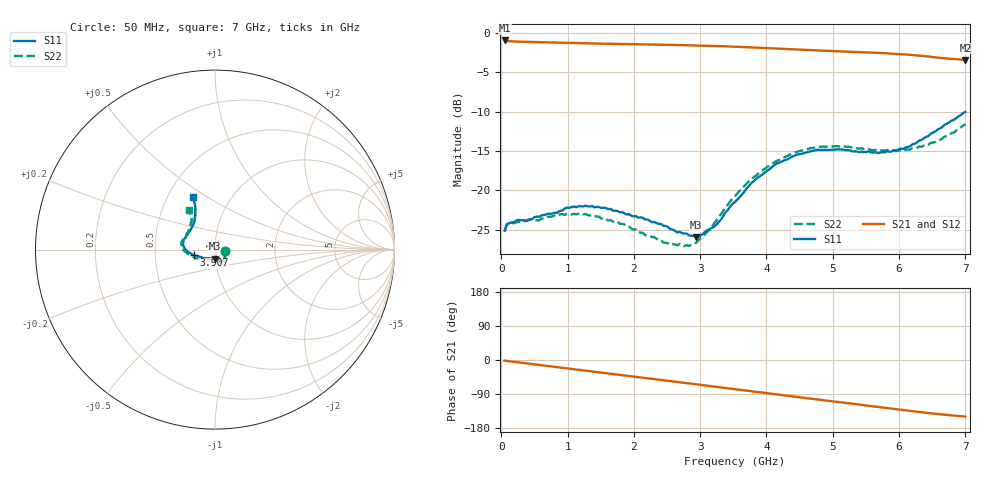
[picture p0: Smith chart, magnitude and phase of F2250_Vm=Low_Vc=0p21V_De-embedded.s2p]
! Integrated Device Technology
! Corporate Headquarters
! 6024 Silver Creek Valley Road
! San Jose, CA 95138  USA
! Phone:  1-408-284-8200
! Toll Free:  1-800-223-1366
! Webpage:  http://www.idt.com/
! Timing and RF Division
! 515 Groton Road, Suite 102
! Westford, MA 01886-6024
! Device:  F2250
! Description: Voltage Variable RF Attenuator
! Frequency:  50.0 -  6000.00 MHz
! Package:  3x3 mm Thin QFN Plastic Package: 16 pin
! Ports:  2 RF, 3 DC
!  Pin  1  = GND
!  Pin  2  = NC
!  Pin  3  = RF1  = Port 1
!  Pin  4  = NC
!  Pin  5  = GND
!  Pin  6  = GND
!  Pin  7  = GND
!  Pin  8  = GND
!  Pin  9  = NC
!  Pin 10  = RF2  = Port 2
!  Pin 11  = NC
!  Pin 12  = GND
!  Pin 13  = GND
!  Pin 14  = VCNTRL
!  Pin 15  = VDD
!  Pin 16  = VMODE
! Vcntrl:  0.210 Volts
! Vmode:  +0.000 Volts
! Vdd:  +3.30  Volts
! Current:  1.105 mA
! Data:  The device was measured on a the F2250 evaluation board which has
!  individual transmission lines to the RF pins.  Data was collected
!  using a calibrated network analyzer.  The evaluation board was
!  de-embedded using a TRL calibration technique.
!  The reference plane is the edge of the package pin.
! Misc:  SN 10
!  Action Tracker AT0258
! Date Measured:  2014-11-26
! Date:  2015-10-15  MJV
! Note:
!  Integrated Device Technology supplies this data as a sample of measured
!  data at the package pin for this product.  Your particular data for this
!  product may vary.
!  Data was taken at 25 degrees C.
!  Integrated Device Technology reserves the right to change this data at anytime.
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# GHz S dB R 50
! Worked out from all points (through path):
!   201 points, 50 MHz to 7 GHz, reference 50 ohm
!   highest |S21| = -0.93 dB at 50 MHz (marker M1); lowest = -3.4 dB at 7 GHz (marker M2)
!   group delay of S21, straight-line fit = 60 ps
!   lowest |S11| = -26.0 dB at 2.934 GHz (marker M3), VSWR 1.11, Z = 49.5 - j4.99 ohm
!   |S11| at or under -10 dB: start of sweep to end of sweep
!   |S22| runs from -27.1 to -11.6 dB; largest |S21 - S12| = 0.00027
!   S11 on the Smith chart (normalised r, x): 50 MHz: 1.12, -0.02; 3.907 GHz: 0.79, -0.05; 7 GHz: 0.67, +0.43
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0.05  -25.11 -9.7  -0.93 -1.8  -0.93 -1.8  -25.23 -10.1
0.08475  -24.29 -9.6  -1.00 -2.5  -0.99 -2.5  -24.34 -9.4
0.15425  -24.07 -11.9  -1.04 -4.0  -1.04 -4.0  -24.11 -11.0
0.57125  -23.35 -30.0  -1.14 -13.1  -1.14 -13.1  -23.82 -30.4
0.884  -22.62 -45.9  -1.21 -19.9  -1.20 -19.9  -23.05 -46.9
1.2315  -22.06 -56.1  -1.28 -27.4  -1.28 -27.4  -23.05 -59.7
1.75275  -22.62 -62.8  -1.37 -38.4  -1.37 -38.4  -23.95 -66.7
2.37825  -24.26 -63.6  -1.46 -51.8  -1.46 -51.8  -26.30 -67.8
2.552  -24.95 -67.8  -1.49 -55.6  -1.49 -55.6  -26.96 -73.3
2.83  -25.72 -83.3  -1.54 -61.7  -1.54 -61.7  -27.08 -92.7
2.93425  -25.97 -92.5  -1.56 -64.0  -1.56 -64.0  -26.70 -101.5
3.21225  -24.62 -122.1  -1.63 -70.1  -1.63 -70.1  -24.17 -127.6
3.525  -21.47 -148.4  -1.72 -77.1  -1.72 -77.1  -20.72 -146.4
3.76825  -19.10 -161.4  -1.81 -82.5  -1.81 -82.5  -18.56 -156.8
3.90725  -18.17 -165.6  -1.87 -85.5  -1.87 -85.5  -17.67 -162.9
4.1505  -16.61 -173.8  -1.97 -90.8  -1.96 -90.8  -16.28 -171.4
4.7065  -14.96 172.2  -2.18 -102.8  -2.18 -102.8  -14.60 175.6
5.15825  -14.82 161.5  -2.33 -112.5  -2.33 -112.5  -14.36 166.5
5.85325  -15.08 138.3  -2.58 -127.5  -2.58 -127.5  -14.99 151.5
6.166  -14.39 127.5  -2.75 -134.3  -2.76 -134.3  -14.80 142.6
6.444  -13.09 119.3  -2.96 -140.1  -2.96 -140.1  -14.18 133.3
7  -10.01 113.0  -3.41 -149.3  -3.41 -149.3  -11.59 123.9
